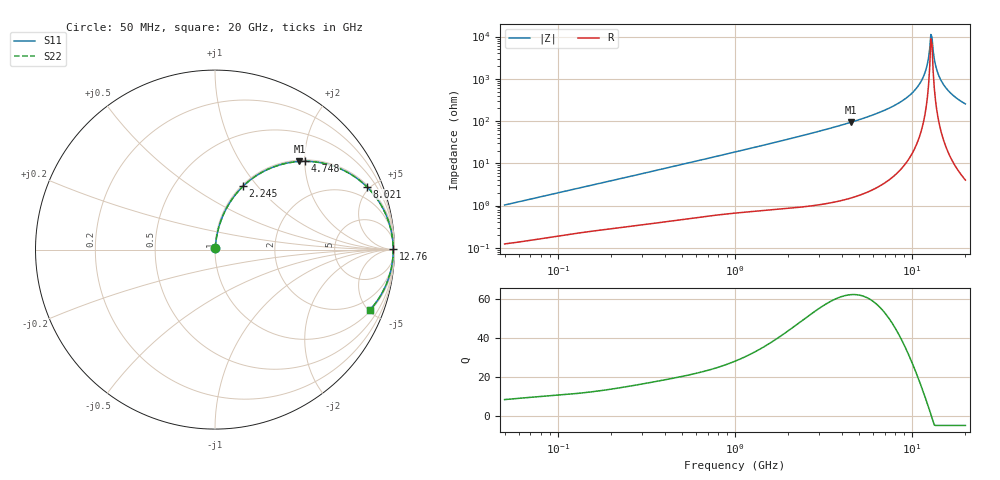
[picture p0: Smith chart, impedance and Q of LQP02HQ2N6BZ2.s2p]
!Murata Part Number: LQP02HQ2N6BZ2
!These Parameters are Measured in Series Mode Connection
!  o--[Z]--o
!Port1  Port2
!  o-------o
!Freq. Start=50[MHz] Stop=20[GHz], 401[Steps]
# Hz S RI R 50
!Freq.(Hz) S11(Real) S11(Imag) S21(Real) S21(Imag) S12(Real) S12(Imag) S22(Real) S22(Imag)
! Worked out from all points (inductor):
!   401 points, 50 MHz to 20 GHz, reference 50 ohm
!   read as one part in series: L = 3.22 nH near 51.52 MHz
!   highest Q = 62.1 at 4.54 GHz (marker M1), where L = 3.3 nH
!   self-resonance near 12.76 GHz
!   S11 on the Smith chart (normalised r, x): 50 MHz: 1.00, +0.02; 2.245 GHz: 1.02, +0.84; 4.748 GHz: 1.03, +2.00; 8.021 GHz: 1.11, +4.77; 12.76 GHz: open; 20 GHz: 1.08, -5.09
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5e7  0.00134 0.0102  0.9987 -0.0102  0.9987 -0.0102  0.00134 0.0102
1.364002e8  0.00299 0.0266  0.997 -0.0266  0.997 -0.0266  0.00299 0.0266
3.721004e8  0.00878 0.0694  0.9912 -0.0694  0.9912 -0.0694  0.00878 0.0694
1e9  0.0391 0.1767  0.9609 -0.1767  0.9609 -0.1767  0.0391 0.1767
2.245319e9  0.1562 0.3526  0.8438 -0.3526  0.8438 -0.3526  0.1562 0.3526
2.728004e9  0.217 0.4028  0.783 -0.4028  0.783 -0.4028  0.217 0.4028
4.539627e9  0.4706 0.4912  0.5294 -0.4912  0.5294 -0.4912  0.4706 0.4912
4.748272e9  0.4993 0.492  0.5007 -0.492  0.5007 -0.492  0.4993 0.492
7.442007e9  0.8004 0.3898  0.1996 -0.3898  0.1996 -0.3898  0.8004 0.3898
8.020766e9  0.8451 0.3509  0.1549 -0.3509  0.1549 -0.3509  0.8451 0.3509
9.600142e9  0.933 0.2344  0.067 -0.2344  0.067 -0.2344  0.933 0.2344
1.098561e10  0.9751 0.1302  0.0249 -0.1302  0.0249 -0.1302  0.9751 0.1302
1.183995e10  0.988 0.0685  0.012 -0.0685  0.012 -0.0685  0.988 0.0685
1.220001e10  0.991 0.0433  0.00904 -0.0433  0.00904 -0.0433  0.991 0.0433
1.257102e10  0.9926 0.018  0.00738 -0.018  0.00738 -0.018  0.9926 0.018
1.276073e10  0.993 0.00537  0.00704 -0.00537  0.00704 -0.00537  0.993 0.00537
1.314879e10  0.9927 -0.02  0.00733 0.02  0.00733 0.02  0.9927 -0.02
1.354865e10  0.9911 -0.0453  0.00892 0.0453  0.00892 0.0453  0.9911 -0.0453
1.396067e10  0.9882 -0.0705  0.0118 0.0705  0.0118 0.0705  0.9882 -0.0705
1.482269e10  0.9786 -0.1201  0.0214 0.1201  0.0214 0.1201  0.9786 -0.1201
1.670968e10  0.9448 -0.2146  0.0552 0.2146  0.0552 0.2146  0.9448 -0.2146
2e10  0.8624 -0.3367  0.1376 0.3367  0.1376 0.3367  0.8624 -0.3367
